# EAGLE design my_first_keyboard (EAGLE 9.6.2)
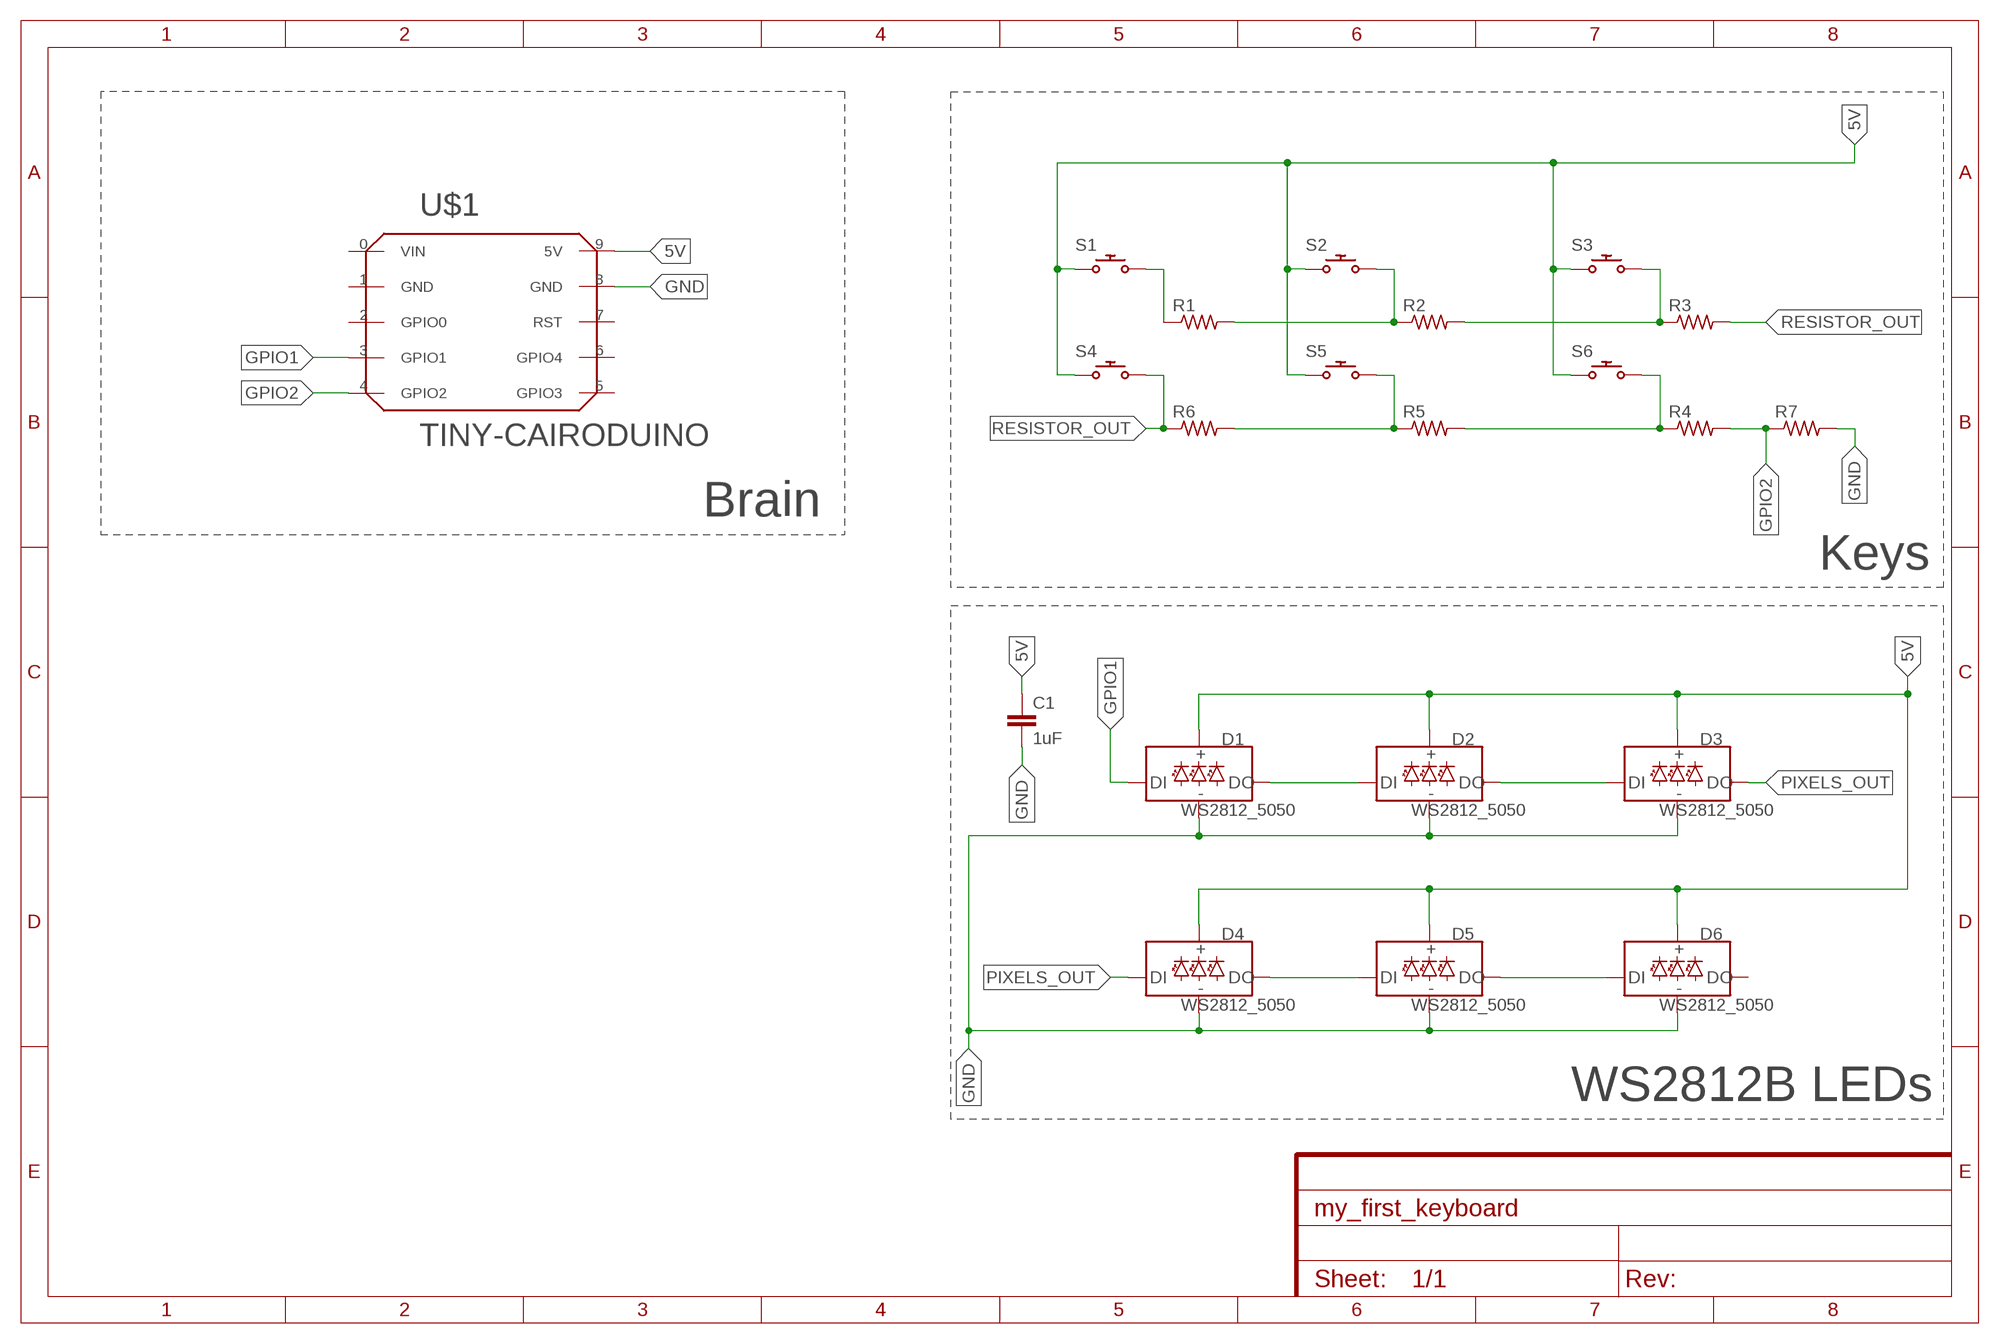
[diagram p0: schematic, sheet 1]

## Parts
C1  1uF  22UF-0805-6.3V-20%  [0805]
D1  WS2812_5050  [WS2812-5X5-4PIN]
D2  WS2812_5050  [WS2812-5X5-4PIN]
D3  WS2812_5050  [WS2812-5X5-4PIN]
D4  WS2812_5050  [WS2812-5X5-4PIN]
D5  WS2812_5050  [WS2812-5X5-4PIN]
D6  WS2812_5050  [WS2812-5X5-4PIN]
R1  R1206FAB  [R1206FAB]
R2  R1206FAB  [R1206FAB]
R3  R1206FAB  [R1206FAB]
R4  R1206FAB  [R1206FAB]
R5  R1206FAB  [R1206FAB]
R6  R1206FAB  [R1206FAB]
R7  R1206FAB  [R1206FAB]
S1  CHERRY_CHERRY_MX  [CHERRY_CHERRY_MX]
S2  CHERRY_CHERRY_MX  [CHERRY_CHERRY_MX]
S3  CHERRY_CHERRY_MX  [CHERRY_CHERRY_MX]
S4  CHERRY_CHERRY_MX  [CHERRY_CHERRY_MX]
S5  CHERRY_CHERRY_MX  [CHERRY_CHERRY_MX]
S6  CHERRY_CHERRY_MX  [CHERRY_CHERRY_MX]
U$1  TINY-CAIRODUINO  [TINY-CAIRODUINO]

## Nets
5V: C1.1 D1.VCC D2.VCC D3.VCC D4.VCC D5.VCC D6.VCC S1.S1 S2.S1 S3.S1 S4.S1 S5.S1 S6.S1 U$1.9(5V)
GND: C1.2 D1.GND D2.GND D3.GND D4.GND D5.GND D6.GND R7.2 U$1.8(GND)
GPIO1: D1.DI U$1.3(GPIO1)
GPIO2: R4.2 R7.1 U$1.4(GPIO2)
N$1: D1.DO D2.DI
N$2: R1.2 R2.1 S2.S2
N$3: R2.2 R3.1 S3.S2
N$4: R5.1 R6.2 S5.S2
N$5: R4.1 R5.2 S6.S2
N$6: D2.DO D3.DI
N$7: R1.1 S1.S2
N$8: D4.DO D5.DI
N$9: D5.DO D6.DI
PIXELS_OUT: D3.DO D4.DI
RESISTOR_OUT: R3.2 R6.1 S4.S2
Unconnected: D6.DO U$1.2(GPIO0) U$1.5(GPIO3) U$1.6(GPIO4) U$1.7(RST)

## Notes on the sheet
- Brain
- Keys
- WS2812B LEDs

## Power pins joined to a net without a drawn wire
GND: U$1.1(GND)
VIN: U$1.0(VIN)

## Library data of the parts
C1 = SparkFun-Capacitors:22UF: 22µF ceramic capacitors; PROD_ID: CAP-08402; VALUE: 22uF
D1-D6 = SparkFun-LED:WS2812: Addressable RGB LED - 1 Wire Common names: WS2812, SK6812, Neopixel, APA-106, etc. SMD LED with built-in controller IC. Color: Red/Green/Blue SparkFun Products: LED-SMD RGB (WS2812) LED - RGB Addressable, PTH, 5mm Diffused (5 Pack) LED - RGB Addressable, PTH, 5mm Clear (5 Pack) Blynk Board -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; PROD_ID: DIO-12503
R1-R7 = fab:R: Resistor (US Symbol)
S1-S6 = Keyboard Library:CHERRY_CHERRY_MX: Cherry keymodule MX; FARNELL: 2292961; MOUSER: 540-MX1A-11NW
U$1 = Cairo:TINY-CAIRODUINO

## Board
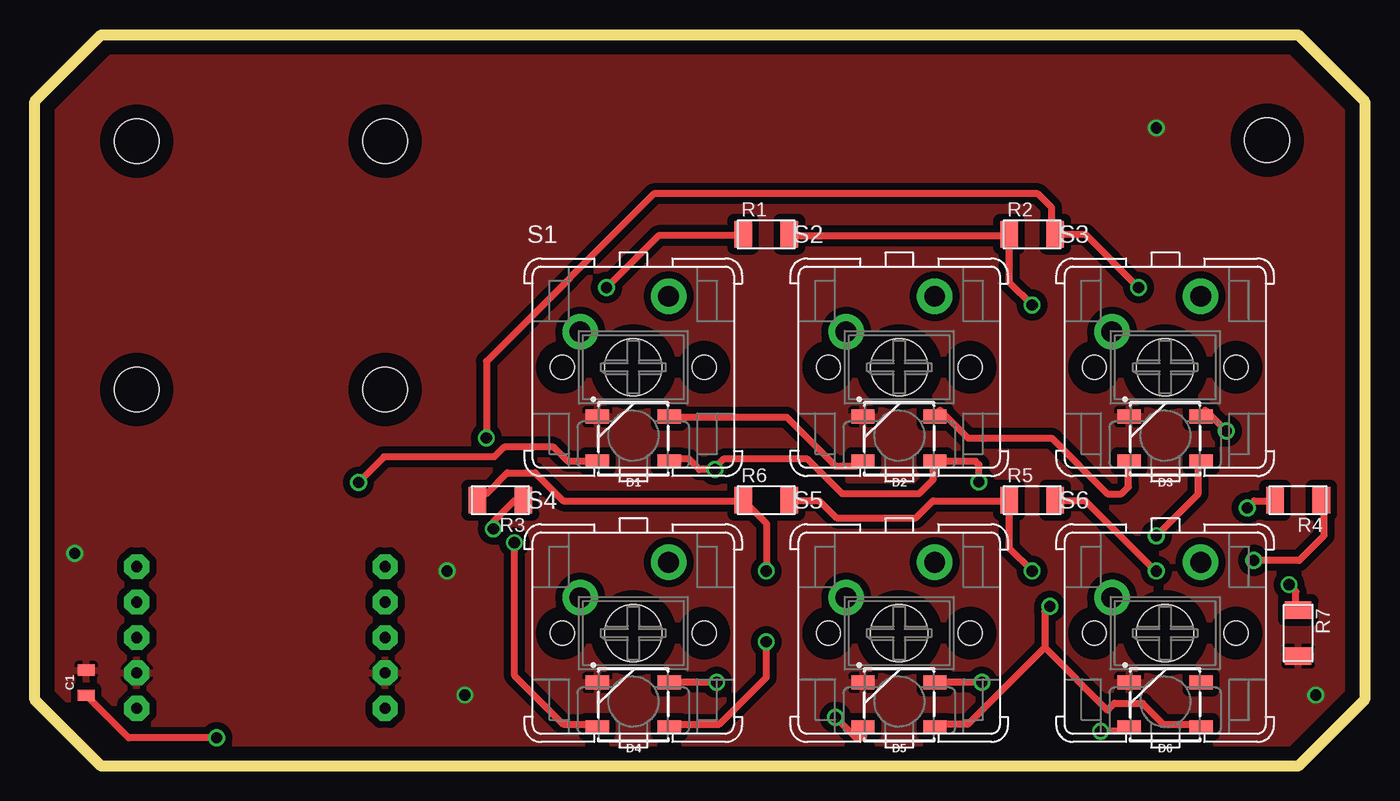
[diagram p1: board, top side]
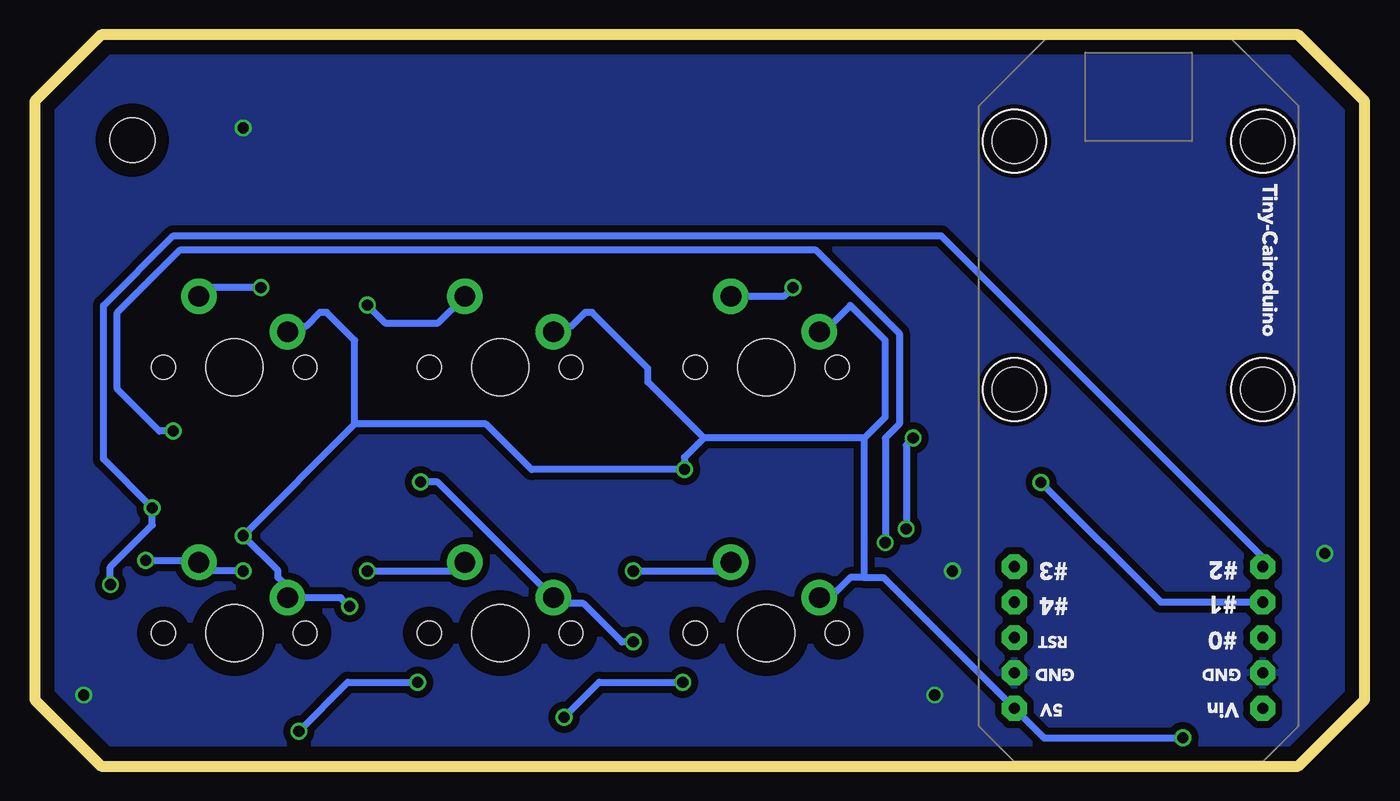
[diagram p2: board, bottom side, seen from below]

Size 95.25 x 52.39 mm. Coordinates in mm from the lower left corner, seen from the top.
Outline: 90.49,0 90.49,0
Outline: 90.49,0 95.25,4.76 95.25,47.62 90.49,52.39 4.76,52.39 0,47.62 0,4.76 4.76,0 90.49,0
Copper layers (1*16): Top 0.035mm / dielectric 1.5mm / Bottom 0.035mm
Design rules "default *": minimum track width 0.5mm, minimum drill 0.8mm, track to track 0.5mm, track to pad 0.5mm, pad to pad 0.5mm, via to via 0.5mm, smd to smd 6mil, copper to edge 40mil, drill to drill 0.5mm, minimum pad ring 10mil, minimum via ring 8mil, stop-mask expansion 4mil, vias tented up to drill 0mil, thermal gap 10mil
Holes 3.2 mm at 88.27,44.83

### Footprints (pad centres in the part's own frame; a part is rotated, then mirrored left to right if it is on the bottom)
0805 = smd 0.8 x 1.2: 1 -0.9,0; 2 0.9,0
WS2812-5X5-4PIN = smd 1.651 x 1: DI 2.577,1.6; DO -2.577,-1.6; GND 2.577,-1.6; VCC -2.577,1.6
R1206FAB = smd 1.27 x 1.905: 1 -1.651,0; 2 1.651,0
CHERRY_CHERRY_MX = drill 1.5 pad 2.54: S1 -3.81,2.54; S2 2.54,5.08 | hole 1.7: -5.08,0; 5.08,0 | hole 4.1: 0,0
TINY-CAIRODUINO = drill 0.8 pad 1.778 octagon: 0 2.54,48.26; 1 2.54,45.72; 2 2.54,43.18; 3 2.54,40.64; 4 2.54,38.1; 5 20.32,38.1; 6 20.32,40.64; 7 20.32,43.18; 8 20.32,45.72; 9 20.32,48.26 | hole 3.2: 20.32,25.4; 2.54,25.4; 2.54,7.62; 20.32,7.62

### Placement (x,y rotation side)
C1  3.68,5.97 90 top
D1  42.86,23.43 180 top
D2  61.91,23.43 180 top
D3  80.96,23.43 180 top
D4  42.86,4.38 180 top
D5  61.91,4.38 180 top
D6  80.96,4.38 180 top
R1  52.39,38.1 0 top
R2  71.44,38.1 0 top
R3  33.34,19.05 180 top
R4  90.49,19.05 180 top
R5  71.44,19.05 0 top
R6  52.39,19.05 0 top
R7  90.49,9.53 270 top
S1  42.86,28.57 0 top
S2  61.91,28.57 0 top
S3  80.96,28.57 0 top
S4  42.86,9.53 0 top
S5  61.91,9.53 0 top
S6  80.96,9.53 0 top
U$1  4.76,52.39 180 bottom

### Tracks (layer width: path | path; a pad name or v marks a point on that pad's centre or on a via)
5V  (via drill 0.8)
  Top 0.5: 72.34,8.5 66.84,3 64.84,3 D5.VCC | 72.34,8.5 72.34,11.06 v72.71,11.43 | 72.34,8.5 76.84,4 77.34,4.5 79.34,4.5 80.84,3 83.34,3 D6.VCC | v80.34,16.5 83.34,19.5 83.34,21.5 D3.VCC | D4.VCC 45.84,3 49.04,3 52.39,6.35 v52.39,8.89 | D1.VCC 45.84,22 46.84,22 47.59,21.25 v48.73,21.25 48.73,21.39 49.34,22 55.34,22 57.84,19.5 63.34,19.5 64.34,20.5 64.34,21.5 D2.VCC 67.39,21.83 67.63,21.59 v67.63,20.35 | v13.02,2.02 6.73,2.02 C1.1
  Bottom 0.5: 72.34,24.5 72.34,30.5 74.34,32.5 74.84,32.5 75.84,31.5 76.84,31.5 S3.S1 | 72.34,24.5 v80.34,16.5 77.84,14 77.84,13.5 76.84,12.5 S6.S1 73.34,12.06 v72.71,11.43 | 35.84,13.5 36.84,13.5 37.84,12.5 38.84,12.5 S4.S1 | 35.84,23.5 34.34,25 34.34,30.5 36.84,33 38.34,31.5 38.84,31.5 S1.S1 | 35.84,13.5 35.84,23.5 | 47.34,23.5 51.34,27.5 51.34,28.5 55.34,32.5 55.84,32.5 56.84,31.5 57.84,31.5 S2.S1 | 35.84,23.5 47.34,23.5 | 47.34,23.5 48.73,22.11 v48.73,21.25 59.66,21.25 62.92,24.5 72.34,24.5 | 35.84,13.5 34.45,13.5 U$1.9 22.97,2.02 v13.02,2.02 | v52.39,8.89 53.21,8.89 55.96,11.64 57.68,11.64 S5.S1 66.39,20.35 v67.63,20.35
GND  (via drill 0.8)
  other vias: 80.33,45.72 91.76,5.08 2.86,15.24 30.8,5.08 29.53,13.97
  pour Top (isolate 0.5): 4.76,0 0,4.76 0,47.62 4.76,52.39 90.49,52.39 95.25,47.62 95.25,4.76 90.49,0
  pour Bottom (isolate 0.5): 4.76,0 0,4.76 0,47.62 4.76,52.39 90.49,52.39 95.25,47.62 95.25,4.76 90.49,0
GPIO1  (via drill 0.8)
  Top 0.5: D1.DI 38.18,21.83 37.15,22.86 33.61,22.86 32.9,22.15 25,22.15 v23.18,20.32
  Bottom 0.5: v23.18,20.32 14.6,11.75 U$1.3
GPIO2  (via drill 0.8)
  Top 0.5: v86.84,18.5 87.34,19 88.34,19 R4.2 | v89.84,13 90.34,12.5 90.34,11.5 R7.1
  Bottom 0.5: v89.84,13 89.84,14.27 86.84,17.27 v86.84,18.5 90.34,22 90.34,33 85.34,38 30.34,38 7.34,15 7.34,14.5 U$1.4
N$1
  Top 0.5: D2.DI 58.84,21.5 57.34,21.5 53.84,25 45.84,25 D1.DO
N$2  (via drill 0.8)
  Top 0.5: R1.2 54.34,38 69.34,38 R2.1 69.79,34.67 v71.44,33.02
  Bottom 0.5: v71.44,33.02 70.17,31.75 66.36,31.75 S2.S2
N$3  (via drill 0.8)
  Top 0.5: v32.84,17 32.84,17.5 34.34,19 34.84,19 R3.1 | v32.34,23.5 32.34,29 44.34,41 71.84,41 72.84,40 72.84,38.5 R2.2 75.25,38.1 v79.06,34.29
  Bottom 0.5: v32.84,17 32.84,23 v32.34,23.5 | v79.06,34.29 82.87,34.29 S3.S2
N$4  (via drill 0.8)
  Top 0.5: R6.2 54.34,19 56.2,19 57.42,17.78 63.12,17.78 64.34,19 69.34,19 R5.1 69.79,15.62 v71.44,13.97
  Bottom 0.5: v71.44,13.97 65.09,13.97 S5.S2
N$5  (via drill 0.8)
  Top 0.5: R5.2 73.34,19 75.25,19 80.28,13.97 v80.33,13.97 | R4.1 92.34,19 92.34,16.5 90.57,14.73 v87.31,14.73
  Bottom 0.5: v80.33,13.97 82.87,13.97 S6.S2 83.63,14.73 v87.31,14.73
N$6
  Top 0.5: D3.DI 78.34,21.5 78.34,20 77.84,19.5 76.84,19.5 72.84,23.5 66.84,23.5 64.84,25.5 D2.DO
N$7  (via drill 0.8)
  Top 0.5: R1.1 50.34,38 44.67,38 v40.96,34.29
  Bottom 0.5: v40.96,34.29 41.59,33.66 S1.S2
N$8  (via drill 0.8)
  Top 0.5: v48.84,6 45.84,6 D4.DO | v57.34,3.5 58.84,2 59.34,2 59.34,2.5 D5.DI
  Bottom 0.5: v48.84,6 54.84,6 v57.34,3.5
N$9  (via drill 0.8)
  Top 0.5: v67.84,6 64.84,6 D5.DO | v76.34,2.5 78.34,2.5 D6.DI
  Bottom 0.5: v67.84,6 72.84,6 v76.34,2.5
PIXELS_OUT  (via drill 0.8)
  Top 0.5: v34.34,16 34.34,6.5 37.84,3 39.84,3 D4.DI | v85.34,24 83.84,25.5 D3.DO
  Bottom 0.5: v34.34,16 34.34,23.5 33.34,24.5 33.34,31 39.34,37 84.84,37 89.34,32.5 89.34,27 86.34,24 v85.34,24
RESISTOR_OUT  (via drill 0.8)
  Top 0.5: R3.2 31.84,19.5 32.34,19.5 33.84,21 35.84,21 37.84,19 50.34,19 R6.1 52.39,17.4 v52.39,13.97
  Bottom 0.5: v52.39,13.97 46.04,13.97 S4.S2

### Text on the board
Measures: Make the pin header cuts bigger to fit the male pin header. Like the Tiny-Cairoduino pin header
